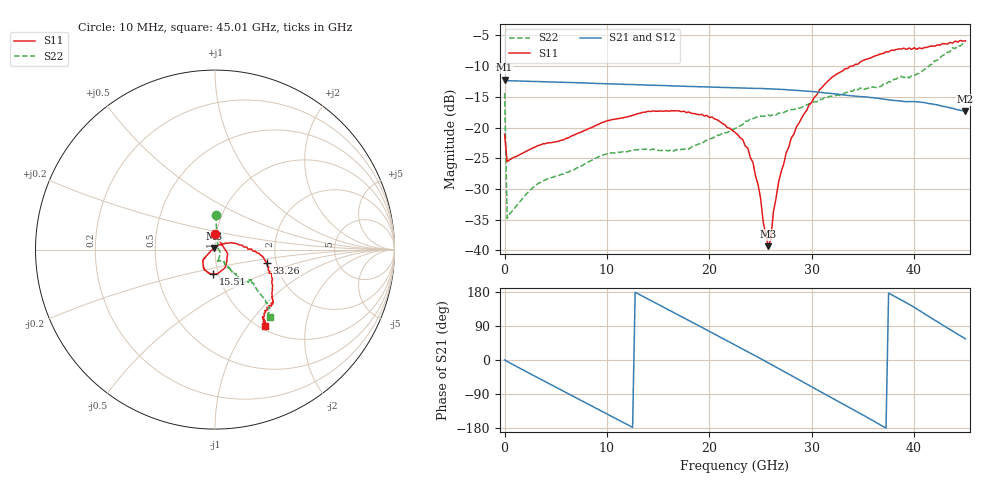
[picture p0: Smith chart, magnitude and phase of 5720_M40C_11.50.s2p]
! Device:  ADRF5720
! Description: 0.5dB LSB GaAs MMIC 6-bit Digital Attenuator
! Frequency:  0.000009 -  40 GHz
! Ports:
!	RF1	= Port 1
!	RF2	= Port 2
! Vdd:  3.3 Volt
! Vss:  -3.3 Volt
! Control:  0/3.3 Volt
! State:  11.50 dB attenuation
! Data:  The device was measured using G-S-G Probes on a matrix board.
!  Data was collected using an calibrated 4 port network analyzer.
!  The reference plane for this measurement is at the launchers.
! Note:  Analog Devices supplies this data as a sample of measured data
!  for this product.  Your particular data for this product may vary.
!  Data was taken at -40 degrees C.
!  Analog Devices reserves the right to change this data at anytime.
# GHZ S DB R 45.0
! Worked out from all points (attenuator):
!   181 points, 10 MHz to 45.01 GHz, reference 45 ohm
!   highest |S21| = -12.20 dB at 10 MHz (marker M1); lowest = -17.3 dB at 45.01 GHz (marker M2)
!   lowest |S11| = -39.3 dB at 25.76 GHz (marker M3), VSWR 1.02, Z = 44.5 + j0.812 ohm
!   |S11| at or under -10 dB: start of sweep to 34.02 GHz
!   |S22| runs from -34.8 to -6.3 dB; largest |S21 - S12| = 0.00089
!   S11 on the Smith chart (normalised r, x): 10 MHz: 0.98, +0.18; 15.51 GHz: 0.95, -0.26; 33.26 GHz: 1.79, -0.30; 45.01 GHz: 1.06, -1.21
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0.01  -21.09 90.0  -12.20 -0.0  -12.22 -0.0  -14.40 88.9
0.26  -25.58 8.2  -12.37 -3.9  -12.39 -4.0  -34.82 24.6
3.26  -22.95 -16.0  -12.52 -46.9  -12.55 -47.0  -29.14 -30.1
7.76  -20.50 -46.4  -12.74 -110.7  -12.76 -110.7  -26.01 -63.3
11.76  -18.34 -70.5  -12.97 -167.2  -12.99 -167.2  -23.93 -77.0
15.26  -17.31 -92.1  -13.15 143.2  -13.17 143.1  -23.75 -77.6
15.51  -17.35 -93.6  -13.16 139.6  -13.18 139.6  -23.73 -76.8
19.01  -17.92 -114.8  -13.35 89.9  -13.37 89.8  -22.66 -60.9
22.76  -21.15 -139.6  -13.54 36.2  -13.57 36.1  -19.99 -55.1
24.26  -25.67 -144.9  -13.62 14.5  -13.64 14.4  -18.56 -54.4
25.01  -31.52 -162.4  -13.64 3.5  -13.66 3.4  -18.14 -53.0
25.26  -35.30 -167.1  -13.65 -0.2  -13.67 -0.4  -18.19 -53.8
25.76  -39.33 122.3  -13.71 -7.6  -13.73 -7.8  -17.96 -53.1
26.01  -38.22 91.3  -13.71 -11.2  -13.74 -11.4  -18.10 -53.1
26.26  -33.75 66.6  -13.73 -15.0  -13.75 -15.2  -17.87 -51.9
26.76  -28.95 51.2  -13.79 -22.4  -13.81 -22.6  -17.65 -52.0
27.51  -24.12 30.6  -13.83 -33.5  -13.85 -33.6  -17.35 -52.9
30.26  -15.07 4.6  -14.17 -74.7  -14.19 -74.8  -15.78 -52.0
33.26  -10.44 -14.8  -14.73 -119.4  -14.75 -119.6  -14.34 -50.3
37.76  -7.41 -40.8  -15.55 173.0  -15.57 172.8  -12.54 -49.3
41.76  -6.70 -53.7  -16.16 109.5  -16.18 109.3  -9.68 -44.0
45.01  -5.89 -56.7  -17.34 55.9  -17.37 55.8  -6.30 -50.9
